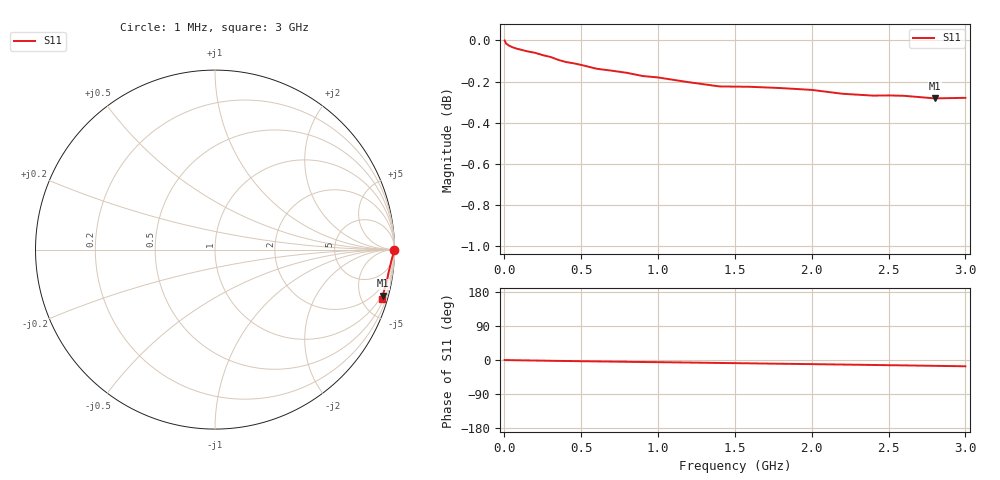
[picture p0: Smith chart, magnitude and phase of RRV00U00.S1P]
! SIEMENS Small Signal Semiconductors
! BA595
! Si PIN Diode in SOD323
! VR = 0 V
! S-Parameters:  July  1992
# GHz  S  MA  R  50
!  f  S11
! GHz  MAG  ANG
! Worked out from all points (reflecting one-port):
!   33 points, 1 MHz to 3 GHz, reference 50 ohm
!   lowest |S11| = -0.3 dB at 2.8 GHz (marker M1), VSWR 61.70, Z = 44.5 - j364 ohm
!   phase of S11 starts at 0 deg and turns -17 deg over the sweep
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0.001  1 0.0
0.003  0.9997 -0.1
0.01  0.9983 -0.2
0.03  0.9971 -0.3
0.05  0.9963 -0.5
0.06  0.996 -0.5
0.08  0.9954 -0.7
0.25  0.9918 -1.7
0.3  0.9908 -2.1
0.35  0.9892 -2.4
0.4  0.988 -2.6
0.5  0.9864 -3.2
0.6  0.9843 -3.7
0.7  0.9832 -4.2
0.8  0.982 -4.8
0.9  0.9803 -5.3
1  0.9795 -5.7
1.2  0.9769 -6.7
1.4  0.9746 -7.8
1.6  0.9744 -8.8
1.8  0.9737 -9.9
2  0.9727 -10.9
2.2  0.9706 -12.0
2.4  0.9696 -13.1
2.5  0.9697 -13.7
2.6  0.9695 -14.2
2.8  0.9681 -15.4
3  0.9684 -16.6
